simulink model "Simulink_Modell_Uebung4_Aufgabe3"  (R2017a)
settings: Solver=VariableStepAuto  StartTime=0.0  StopTime=2  RelTol=1e-3
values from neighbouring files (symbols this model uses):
  Km_torque = 0.11    [RobotikI_Uebung4.m]
libraries: cstblocks x2, simulink x2

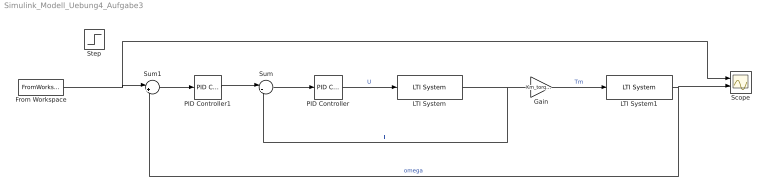
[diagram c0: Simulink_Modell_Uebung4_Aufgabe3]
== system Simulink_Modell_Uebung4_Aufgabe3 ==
  From Workspace : FromWorkspace  VariableName=qdv  SampleTime=0
  Gain : Gain  Gain=Km_torque
  LTI System : cstblocks/LTI System  sys=motor  IC=[]
  LTI System1 : cstblocks/LTI System  sys=robotarm  IC=[]
  PID Controller : simulink/Continuous/PID Controller  Controller=PI  TimeDomain=Continuous-time  SampleTime=-1  IntegratorMethod=Forward Euler  FilterMethod=Forward Euler  Form=Parallel  UseFilter=on  ControllerParametersSource=internal  P=0.503194131871708  I=147.813276237314  D=0  N=100  InitialConditionSource=internal  InitialConditionForIntegrator=0  InitialConditionForFilter=0  ExternalReset=none  LimitOutput=off  UpperSaturationLimit=inf  LowerSaturationLimit=-inf  LinearizeAsGain=on  AntiWindupMode=none  Kb=1  TrackingMode=off  Kt=1  PParamMin=[]  PParamMax=[]  IParamMin=[]  IParamMax=[]  DParamMin=[]  DParamMax=[]  NParamMin=[]  NParamMax=[]  KbParamMin=[]  KbParamMax=[]  KtParamMin=[]  KtParamMax=[]  POutMin=[]  POutMax=[]  IOutMin=[]  IOutMax=[]  DOutMin=[]  DOutMax=[]  NOutMin=[]  NOutMax=[]  KbOutMin=[]  KbOutMax=[]  KtOutMin=[]  KtOutMax=[]  IntegratorOutMin=[]  IntegratorOutMax=[]  FilterOutMin=[]  FilterOutMax=[]  SumOutMin=[]  SumOutMax=[]  SumI1OutMin=[]  SumI1OutMax=[]  SumI2OutMin=[]  SumI2OutMax=[]  SumI3OutMin=[]  SumI3OutMax=[]  SumDOutMin=[]  SumDOutMax=[]  SaturationOutMin=[]  SaturationOutMax=[]  IntegratorContinuousStateAttributes=''  IntegratorStateMustResolveToSignalObject=off  IntegratorRTWStateStorageClass=Auto  FilterContinuousStateAttributes=''  FilterStateMustResolveToSignalObject=off  FilterRTWStateStorageClass=Auto  DifferentiatorICPrevScaledInput=0  DifferentiatorOutMin=[]  DifferentiatorOutMax=[]  InitialConditionSetting=State (most efficient)
  PID Controller1 : simulink/Continuous/PID Controller  Controller=PI  TimeDomain=Continuous-time  SampleTime=-1  IntegratorMethod=Forward Euler  FilterMethod=Forward Euler  Form=Parallel  UseFilter=on  ControllerParametersSource=internal  P=0.017847069208424  I=0.30761203968017  D=0  N=100  InitialConditionSource=internal  InitialConditionForIntegrator=0  InitialConditionForFilter=0  ExternalReset=none  LimitOutput=off  UpperSaturationLimit=inf  LowerSaturationLimit=-inf  LinearizeAsGain=on  AntiWindupMode=none  Kb=1  TrackingMode=off  Kt=1  PParamMin=[]  PParamMax=[]  IParamMin=[]  IParamMax=[]  DParamMin=[]  DParamMax=[]  NParamMin=[]  NParamMax=[]  KbParamMin=[]  KbParamMax=[]  KtParamMin=[]  KtParamMax=[]  POutMin=[]  POutMax=[]  IOutMin=[]  IOutMax=[]  DOutMin=[]  DOutMax=[]  NOutMin=[]  NOutMax=[]  KbOutMin=[]  KbOutMax=[]  KtOutMin=[]  KtOutMax=[]  IntegratorOutMin=[]  IntegratorOutMax=[]  FilterOutMin=[]  FilterOutMax=[]  SumOutMin=[]  SumOutMax=[]  SumI1OutMin=[]  SumI1OutMax=[]  SumI2OutMin=[]  SumI2OutMax=[]  SumI3OutMin=[]  SumI3OutMax=[]  SumDOutMin=[]  SumDOutMax=[]  SaturationOutMin=[]  SaturationOutMax=[]  IntegratorContinuousStateAttributes=''  IntegratorStateMustResolveToSignalObject=off  IntegratorRTWStateStorageClass=Auto  FilterContinuousStateAttributes=''  FilterStateMustResolveToSignalObject=off  FilterRTWStateStorageClass=Auto  DifferentiatorICPrevScaledInput=0  DifferentiatorOutMin=[]  DifferentiatorOutMax=[]  InitialConditionSetting=State (most efficient)
  Scope : Scope  NumInputPorts=2
  Step : Step  After=100  SampleTime=0
  Sum : Sum  Inputs=|+-
  Sum1 : Sum  Inputs=|+-
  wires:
  PID Controller/1 -> LTI System/1  "U"
  LTI System/1 -> Sum/2, Gain/1  "I"
  Sum/1 -> PID Controller/1
  Gain/1 -> LTI System1/1  "Tm"
  LTI System1/1 -> Sum1/2, Scope/2  "omega"
  Sum1/1 -> PID Controller1/1
  PID Controller1/1 -> Sum/1
  From Workspace/1 -> Scope/1, Sum1/1
